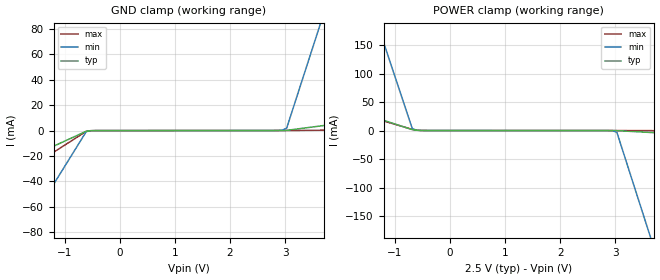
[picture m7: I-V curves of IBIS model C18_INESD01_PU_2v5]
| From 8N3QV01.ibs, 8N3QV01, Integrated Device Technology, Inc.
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[Model] C18_INESD01_PU_2v5
Model_type   Input
Polarity   Non-Inverting
Vinl = 0.7V
Vinh = 1.7V
|   typ   min   max
C_comp   2pF   1.5pF   2.5pF
|   typ   min   max
[Voltage range]   2.5V   2.375V   2.625V
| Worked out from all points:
|   GND clamp passes 1 mA (typ) near -0.63 V on its own axis
|   POWER clamp passes 1 mA (typ) near -0.64 V on its own axis
[GND_clamp]
|Voltage   I (typ)   I (min)   I (max)
-2.5V     -38.24mA   -133.4mA   -53.3mA
-1.818V   -24.68mA   -85.68mA   -34.35mA
-1.742V   -23.17mA   -80.38mA   -32.24mA
-606.1mV  -561.5uA   -857.1uA   -660.6uA
-454.5mV  -73.25uA   -73.73uA   -74.15uA
2.955V    25.53uA    378.8uA    7.086uA
3.03V     127.1uA    1.838mA    10.62uA
3.561V    3.13mA     73.08mA    203.5uA
3.636V    3.559mA    83.25mA    231uA
5V        11.28mA    266.4mA    726.9uA
[Power_clamp]
|Voltage   I (typ)   I (min)   I (max)
-2.5V     58.46mA    531.7mA    53.33mA
-1.364V   22.93mA    201.5mA    21.27mA
-1.288V   20.56mA    179.5mA    19.14mA
-681.8mV  1.609mA    3.381mA    2.038mA
-606.1mV  556uA      651uA      681uA
-454.5mV  25.53uA    29.97uA    21.46uA
2.955V    -73.25uA   -468uA     -62.81uA
3.03V     -155.4uA   -2.979mA   -65.88uA
3.561V    -2.998mA   -162.9mA   -211.6uA
3.636V    -3.404mA   -185.7mA   -232.4uA
5V        -10.71mA   -596.8mA   -607uA
